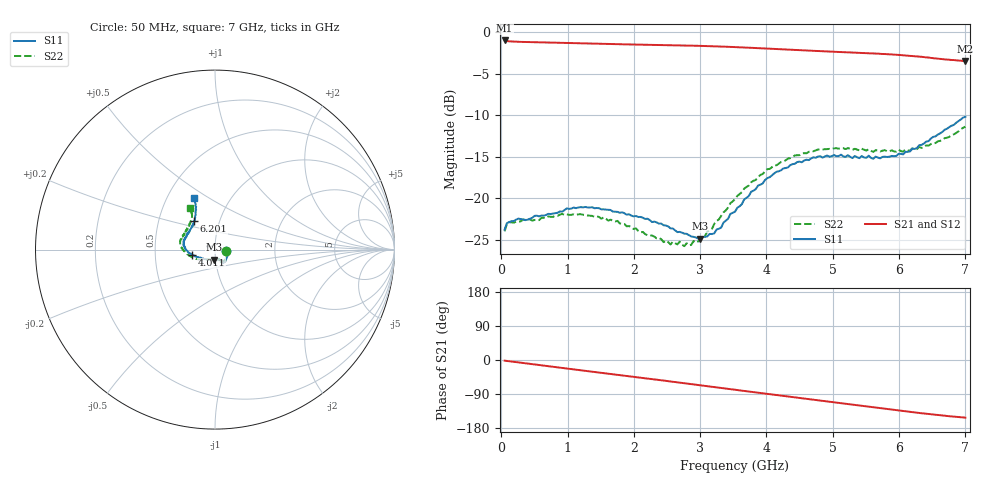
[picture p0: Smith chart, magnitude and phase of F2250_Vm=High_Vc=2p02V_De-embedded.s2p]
! Integrated Device Technology
! Corporate Headquarters
! 6024 Silver Creek Valley Road
! San Jose, CA 95138  USA
! Phone:  1-408-284-8200
! Toll Free:  1-800-223-1366
! Webpage:  http://www.idt.com/
! Timing and RF Division
! 515 Groton Road, Suite 102
! Westford, MA 01886-6024
! Device:  F2250
! Description: Voltage Variable RF Attenuator
! Frequency:  50.0 -  6000.00 MHz
! Package:  3x3 mm Thin QFN Plastic Package: 16 pin
! Ports:  2 RF, 3 DC
!  Pin  1  = GND
!  Pin  2  = NC
!  Pin  3  = RF1  = Port 1
!  Pin  4  = NC
!  Pin  5  = GND
!  Pin  6  = GND
!  Pin  7  = GND
!  Pin  8  = GND
!  Pin  9  = NC
!  Pin 10  = RF2  = Port 2
!  Pin 11  = NC
!  Pin 12  = GND
!  Pin 13  = GND
!  Pin 14  = VCNTRL
!  Pin 15  = VDD
!  Pin 16  = VMODE
! Vcntrl:  2.020 Volts
! Vmode:  +3.300 Volts
! Vdd:  +3.30  Volts
! Current:  1.319 mA
! Data:  The device was measured on a the F2250 evaluation board which has
!  individual transmission lines to the RF pins.  Data was collected
!  using a calibrated network analyzer.  The evaluation board was
!  de-embedded using a TRL calibration technique.
!  The reference plane is the edge of the package pin.
! Misc:  SN 10
!  Action Tracker AT0258
! Date Measured:  2014-11-26
! Date:  2015-10-15  MJV
! Note:
!  Integrated Device Technology supplies this data as a sample of measured
!  data at the package pin for this product.  Your particular data for this
!  product may vary.
!  Data was taken at 25 degrees C.
!  Integrated Device Technology reserves the right to change this data at anytime.
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# GHz S dB R 50
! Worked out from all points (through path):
!   201 points, 50 MHz to 7 GHz, reference 50 ohm
!   highest |S21| = -1.01 dB at 50 MHz (marker M1); lowest = -3.5 dB at 7 GHz (marker M2)
!   group delay of S21, straight-line fit = 61.1 ps
!   lowest |S11| = -24.9 dB at 3.004 GHz (marker M3), VSWR 1.12, Z = 49.3 - j5.62 ohm
!   |S11| at or under -10 dB: start of sweep to end of sweep
!   |S22| runs from -25.8 to -11.4 dB; largest |S21 - S12| = 0.0019
!   S11 on the Smith chart (normalised r, x): 50 MHz: 1.14, -0.02; 4.011 GHz: 0.77, -0.04; 6.201 GHz: 0.75, +0.25; 7 GHz: 0.68, +0.43
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0.05  -23.79 -8.7  -1.01 -1.8  -1.01 -1.8  -23.99 -9.4
0.08475  -23.01 -8.0  -1.09 -2.5  -1.09 -2.5  -23.11 -8.4
0.1195  -22.88 -8.6  -1.12 -3.3  -1.12 -3.2  -22.92 -8.0
0.91875  -21.63 -44.3  -1.31 -21.0  -1.31 -21.1  -21.90 -47.5
1.2315  -21.11 -52.1  -1.38 -27.9  -1.38 -27.9  -22.00 -57.9
1.75275  -21.65 -58.9  -1.47 -39.1  -1.47 -39.1  -22.74 -65.8
2.37825  -23.07 -59.7  -1.56 -52.7  -1.56 -52.8  -24.79 -69.6
2.552  -23.63 -63.9  -1.58 -56.6  -1.58 -56.6  -25.58 -76.1
2.691  -24.06 -70.5  -1.61 -59.7  -1.61 -59.7  -25.24 -83.1
2.7605  -24.28 -72.4  -1.62 -61.2  -1.62 -61.3  -25.78 -87.2
3.00375  -24.89 -93.7  -1.67 -66.7  -1.67 -66.7  -24.76 -108.8
3.21225  -24.24 -115.5  -1.71 -71.4  -1.71 -71.4  -23.10 -127.1
3.525  -21.64 -143.5  -1.81 -78.5  -1.81 -78.5  -20.13 -145.8
3.76825  -19.23 -158.0  -1.90 -84.0  -1.90 -84.0  -18.10 -157.2
4.0115  -17.59 -167.5  -2.00 -89.4  -2.00 -89.4  -16.51 -167.0
4.4285  -15.86 -179.7  -2.16 -98.6  -2.16 -98.6  -14.85 -179.7
4.7065  -15.08 173.0  -2.26 -104.8  -2.26 -104.8  -14.36 174.3
5.054  -14.94 164.7  -2.39 -112.4  -2.38 -112.5  -13.97 167.0
5.85325  -15.01 138.3  -2.68 -129.9  -2.69 -130.0  -14.38 148.0
6.20075  -14.06 126.2  -2.89 -137.6  -2.89 -137.7  -13.99 138.8
6.54825  -12.57 117.7  -3.16 -144.6  -3.17 -144.8  -13.37 127.4
7  -10.20 112.4  -3.49 -152.0  -3.50 -152.1  -11.40 121.1
